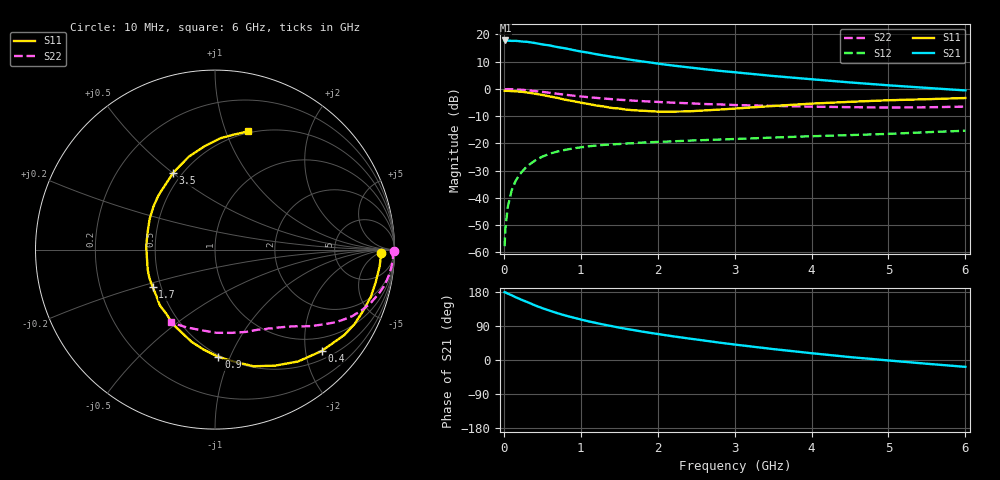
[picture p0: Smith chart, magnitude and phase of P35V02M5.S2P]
! SIEMENS Small Signal Semiconductors
! BFP181
! Si NPN RF Bipolar Junction Transistor in SOT143
! VCE = 5 V  IC = 2.5 mA
! Common Emitter S-Parameters:  March  1996
# GHz  S  MA  R  50
!  f  S11  S21  S12  S22
! GHz  MAG  ANG  MAG  ANG  MAG  ANG  MAG  ANG
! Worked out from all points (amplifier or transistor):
!   36 points, 10 MHz to 6 GHz, reference 50 ohm
!   highest |S21| = 17.8 dB at 20 MHz (marker M1)
!   |S21| within 3 dB of that: start of sweep to 817.1 MHz
!   unconditionally stable (mu >= 1): 2.332 GHz to end of sweep
!   at 250 MHz: K = 0.14, MSG = 23.7 dB, |S12| = -29.9 dB
!   at 1.4 GHz: K = 0.69, MSG = 16.1 dB, |S12| = -20.3 dB
!   at 6 GHz: K = 1.12, MAG = 5.3 dB, |S12| = -15.3 dB
!   S11 on the Smith chart (normalised r, x): 10 MHz: 23, -7; 400 MHz: 0.68, -2.33; 900 MHz: 0.49, -0.91; 1.7 GHz: 0.45, -0.23; 3.5 GHz: 0.45, +0.50; 6 GHz: 0.48, +1.19
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0.01  0.9235 -1.3  7.741 179.0  0.0013 82.2  0.9954 -0.4
0.02  0.9242 -2.5  7.772 178.5  0.0027 86.5  0.9874 -1.0
0.05  0.9225 -5.5  7.741 175.3  0.0067 92.4  0.993 -2.6
0.1  0.9139 -11.3  7.626 170.9  0.0135 83.4  0.9892 -5.1
0.15  0.9073 -16.8  7.652 166.1  0.0201 79.5  0.982 -7.7
0.25  0.8815 -28.0  7.395 157.2  0.0319 73.2  0.9615 -12.5
0.3  0.8632 -33.5  7.338 153.4  0.0378 70.1  0.9475 -14.7
0.4  0.8197 -43.6  6.989 144.5  0.048 64.6  0.9166 -19.0
0.5  0.7764 -53.4  6.582 136.8  0.0572 59.4  0.8833 -22.6
0.6  0.7274 -62.8  6.279 129.8  0.065 54.9  0.8494 -25.9
0.7  0.6839 -71.8  5.861 123.4  0.0712 50.8  0.814 -28.7
0.8  0.6333 -80.2  5.567 117.3  0.0763 47.2  0.7833 -31.1
0.9  0.5984 -88.2  5.199 112.1  0.081 44.4  0.7546 -33.1
1.1  0.5298 -104.3  4.632 102.0  0.0886 39.4  0.7061 -36.7
1.4  0.4487 -127.3  3.905 89.5  0.0962 33.9  0.651 -41.1
1.7  0.4057 -148.8  3.353 78.5  0.1014 30.7  0.6079 -44.7
2.2  0.3839 177.2  2.689 62.5  0.1093 26.7  0.5599 -50.8
2.8  0.4184 145.1  2.155 45.9  0.118 23.4  0.5209 -58.8
3.5  0.4871 118.7  1.731 28.9  0.1282 20.6  0.4893 -69.7
4.5  0.5806 95.4  1.318 7.7  0.1423 16.4  0.4636 -89.1
5.5  0.6486 80.8  1.047 -9.9  0.1608 13.7  0.4614 -110.2
6  0.6825 74.6  0.94 -18.1  0.1711 11.2  0.4737 -121.1
